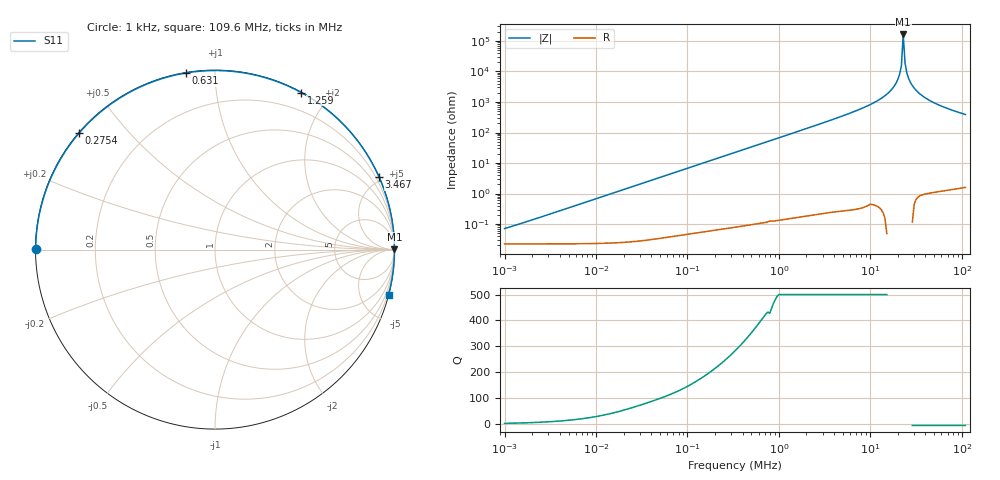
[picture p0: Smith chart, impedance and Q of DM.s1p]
! EM Consulting and Software
! Touchstone file was created on 2026-03-09  16:25:52
# HZ S RI R 50.0000
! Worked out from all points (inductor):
!   253 points, 1 kHz to 109.6 MHz, reference 50 ohm
!   read as one part to ground: L = 10.8 uH near 1.047 kHz
!   highest |Z| = 163 kohm at 22.91 MHz (marker M1)
!   self-resonance near 22.91 MHz
!   S11 on the Smith chart (normalised r, x): 1 kHz: 0.00, +0.00; 275.4 kHz: 0.00, +0.37; 631 kHz: 0.00, +0.85; 1.259 MHz: 0.00, +1.69; 3.467 MHz: 0.00, +4.75; 109.6 MHz: 0.03, -7.80
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1000  -0.9991 0.0027
4365.158  -0.999 0.0118
18197.01  -0.9978 0.0491
41686.94  -0.9924 0.112
79432.82  -0.9758 0.2112
114815.4  -0.9516 0.3012
165958.7  -0.9032 0.4241
218776.2  -0.8389 0.5398
275422.9  -0.7574 0.6491
331131.1  -0.6682 0.7405
380189.4  -0.5851 0.8077
457088.2  -0.4518 0.8891
630957.3  -0.1643 0.9839
724436  -0.0278 0.9973
870963.6  0.1549 0.9858
1047129  0.3279 0.9428
1258925  0.4817 0.8746
1445440  0.581 0.8123
1737801  0.6908 0.7215
2187762  0.7942 0.6063
2754229  0.8663 0.4984
3467369  0.9148 0.4028
6025596  0.9736 0.2277
1.047129e7  0.9936 0.1126
2.290868e7  1 0.000612
2.630268e7  0.9999 -0.0172
5.754399e7  0.9915 -0.1286
1.096478e8  0.9667 -0.252
